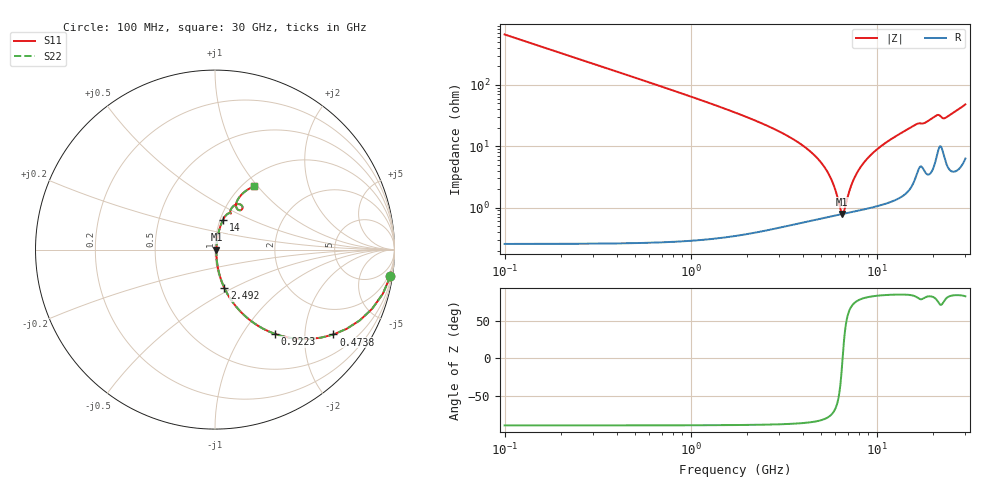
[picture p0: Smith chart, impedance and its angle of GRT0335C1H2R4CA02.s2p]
!Murata Part Number: GRT0335C1H2R4CA02
!These Parameters are Measured in Series Mode Connection
!Data Generated on Jun 19, 2026
!  o--ll--o
!Port1  Port2
!  o------o
!Operation Temp=25[degC], DC Bias Voltage=0[V]
!Freq. Start=100[MHz] Stop=30[GHz] 401[Steps]
# Hz S RI R 50
!Freq.(Hz) S11(Real) S11(Imag) S21(Real) S21(Imag) S12(Real) S12(Imag) S22(Real) S22(Imag)
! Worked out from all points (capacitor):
!   401 points, 100 MHz to 30 GHz, reference 50 ohm
!   read as one part in series: C = 2.4 pF near 249.5 MHz
!   lowest |Z| = 792 mohm at 6.529 GHz (marker M1)
!   series resonance near 6.563 GHz, so ESL is about 240 pH
!   S11 on the Smith chart (normalised r, x): 100 MHz: 1, -13; 473.8 MHz: 1.01, -2.78; 922.2 MHz: 1.01, -1.41; 2.492 GHz: 1.01, -0.45; 14 GHz: 1.03, +0.35; 30 GHz: 1.13, +0.96
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1e8  0.9777 -0.1475  0.0223 0.1475  0.0223 0.1475  0.9777 -0.1475
3.2425e8  0.8059 -0.3948  0.1941 0.3948  0.1941 0.3948  0.8059 -0.3948
4.7375e8  0.6593 -0.473  0.3407 0.473  0.3407 0.473  0.6593 -0.473
9.2225e8  0.3321 -0.469  0.6679 0.469  0.6679 0.469  0.3321 -0.469
1.52025e9  0.1469 -0.3501  0.8531 0.3501  0.8531 0.3501  0.1469 -0.3501
2.492e9  0.0524 -0.2137  0.9476 0.2137  0.9476 0.2137  0.0524 -0.2137
4.21125e9  0.0141 -0.0899  0.9859 0.0899  0.9859 0.0899  0.0141 -0.0899
5.10825e9  0.00917 -0.0498  0.9908 0.0498  0.9908 0.0498  0.00917 -0.0498
5.781e9  0.00785 -0.025  0.9922 0.025  0.9922 0.025  0.00785 -0.025
6.5285e9  0.00779 -0.00104  0.9922 0.00104  0.9922 0.00104  0.00779 -0.00104
6.678e9  0.00791 0.00341  0.9921 -0.00341  0.9921 -0.00341  0.00791 0.00341
7.35075e9  0.0089 0.0223  0.9911 -0.0223  0.9911 -0.0223  0.0089 0.0223
7.874e9  0.0101 0.036  0.9899 -0.036  0.9899 -0.036  0.0101 0.036
8.84575e9  0.0131 0.0594  0.9869 -0.0594  0.9869 -0.0594  0.0131 0.0594
1.01165e10  0.0183 0.0875  0.9817 -0.0875  0.9817 -0.0875  0.0183 0.0875
1.40035e10  0.0436 0.1635  0.9564 -0.1635  0.9564 -0.1635  0.0436 0.1635
1.505e10  0.0548 0.1829  0.9452 -0.1829  0.9452 -0.1829  0.0548 0.1829
2.005825e10  0.1092 0.2473  0.8908 -0.2473  0.8908 -0.2473  0.1092 0.2473
2.1329e10  0.147 0.2479  0.853 -0.2479  0.853 -0.2479  0.147 0.2479
2.289875e10  0.126 0.224  0.874 -0.224  0.874 -0.224  0.126 0.224
2.50665e10  0.1262 0.2774  0.8738 -0.2774  0.8738 -0.2774  0.1262 0.2774
3e10  0.2173 0.3516  0.7827 -0.3516  0.7827 -0.3516  0.2173 0.3516
